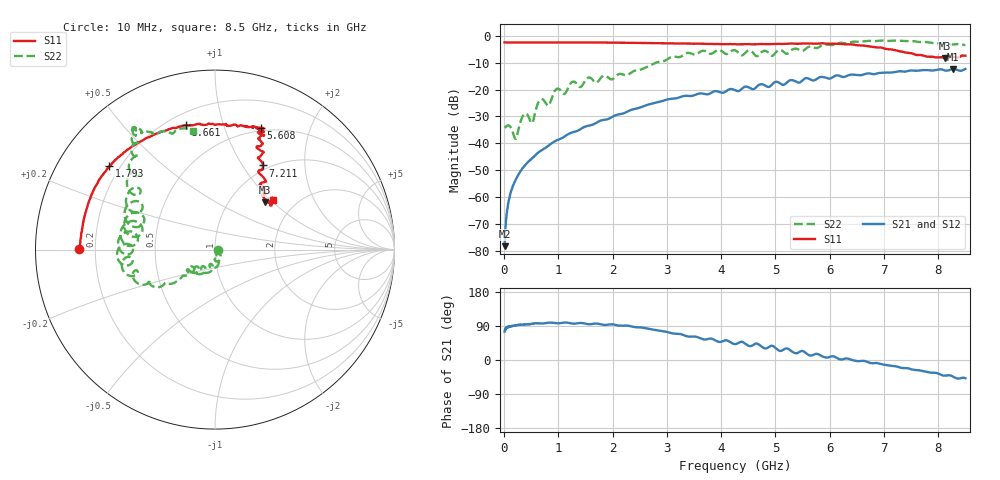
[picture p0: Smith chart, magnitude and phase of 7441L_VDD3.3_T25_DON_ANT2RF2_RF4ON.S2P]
!Agilent Technologies,E5071C,MY46417908,A.11.23
!Date: Mon May 03 19:54:44 2021
!Data & Calibration Information:
!Freq	S11:SOLT2(ON)	S21:SOLT2(ON)	S12:SOLT2(ON)	S22:SOLT2(ON)
!PortZ  Port1:50+j0  Port2:50+j0
!Above PortZ is port z conversion or system Z0 setting when saving the data.
!When reading, reference impedance value at option line is always used.
# Hz S dB R 50
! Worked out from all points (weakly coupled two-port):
!   1601 points, 10 MHz to 8.5 GHz, reference 50 ohm
!   highest |S21| = -12.30 dB at 8.277 GHz (marker M1); lowest = -78.2 dB at 10 MHz (marker M2)
!   lowest |S11| = -8.3 dB at 8.118 GHz (marker M3), VSWR 2.25, Z = 72.6 + j44.9 ohm
!   |S11| at or under -10 dB: nowhere
!   |S22| runs from -38.3 to -1.7 dB; largest |S21 - S12| = 0.0035
!   S11 on the Smith chart (normalised r, x): 10 MHz: 0.14, +0.00; 1.793 GHz: 0.16, +0.34; 3.661 GHz: 0.27, +0.76; 5.608 GHz: 0.47, +1.33; 7.211 GHz: 0.94, +1.24; 8.5 GHz: 1.53, +1.04
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1e7  -2.43 179.7  -78.24 75.2  -78.64 63.0  -34.24 -2.0
6.836875e7  -2.47 178.2  -63.30 88.2  -63.56 86.3  -33.33 -20.7
1.214312e8  -2.48 176.8  -58.44 89.0  -58.49 89.0  -34.03 -40.0
2.169438e8  -2.50 174.3  -53.44 91.1  -53.48 91.4  -38.31 -29.0
3.28375e8  -2.50 171.7  -49.64 93.3  -49.58 93.3  -30.49 -32.6
5.140938e8  -2.50 167.1  -45.56 96.0  -45.57 95.5  -32.42 -61.0
6.520562e8  -2.49 164.0  -43.08 96.5  -43.06 96.4  -24.09 -63.4
8.1655e8  -2.49 160.4  -40.93 98.3  -40.90 98.1  -25.97 -82.9
9.704312e8  -2.46 157.1  -38.87 97.0  -38.85 96.9  -19.74 -92.6
1.426769e9  -2.46 148.5  -34.47 97.9  -34.45 97.8  -18.82 -118.4
1.7929e9  -2.51 141.7  -31.45 93.8  -31.43 94.0  -15.43 -130.1
2.843538e9  -2.75 121.1  -24.63 77.9  -24.64 78.0  -9.72 -144.9
3.6607e9  -2.95 103.3  -21.48 54.8  -21.50 54.9  -5.57 -167.8
4.255e9  -3.11 90.6  -20.23 42.0  -20.25 41.8  -5.38 173.4
4.939506e9  -3.04 78.6  -18.06 37.5  -18.01 37.6  -7.44 159.3
5.608094e9  -2.82 69.4  -15.87 13.5  -15.87 13.8  -4.14 142.2
5.671769e9  -2.88 70.8  -16.51 12.1  -16.50 12.1  -4.06 136.1
7.088538e9  -5.00 64.7  -13.61 -14.7  -13.60 -14.4  -1.90 124.0
7.210581e9  -5.36 60.3  -13.42 -16.5  -13.41 -16.3  -1.74 123.8
8.11795e9  -8.29 43.2  -12.86 -41.3  -12.77 -41.4  -2.90 113.1
8.277138e9  -7.80 39.1  -12.30 -44.1  -12.19 -44.2  -3.22 109.5
8.5e9  -7.39 40.5  -12.30 -48.1  -12.21 -47.7  -3.44 100.7
